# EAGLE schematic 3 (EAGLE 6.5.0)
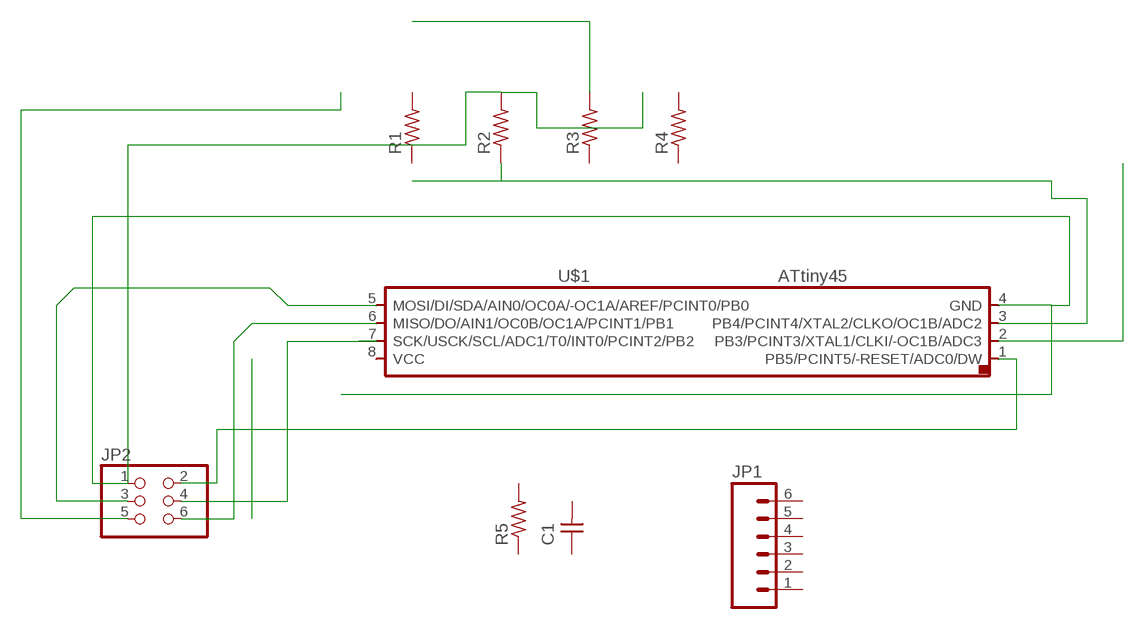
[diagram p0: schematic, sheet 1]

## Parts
C1  UNPOLARIZED_CAPACITOR1206  [1206]
JP1  M06SMD  [1X06-SMD]
JP2  PINHD-2X3-SMD  [2X03SMD]
R1  RESISTOR1206  [1206]
R2  RESISTOR1206  [1206]
R3  RESISTOR1206  [1206]
R4  RESISTOR1206  [1206]
R5  RESISTOR1206  [1206]
U$1  ATTINY45SI  [SOIC8]

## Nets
N$1: JP2.3 U$1.5(MOSI/DI/SDA/AIN0/OC0A/-OC1A/AREF/PCINT0/PB0)
N$2: JP2.5
N$3: JP2.2 U$1.1(PB5/PCINT5/-RESET/ADC0/DW)
N$5: JP2.4 U$1.7(SCK/USCK/SCL/ADC1/T0/INT0/PCINT2/PB2)
N$6: JP2.6 U$1.6(MISO/DO/AIN1/OC0B/OC1A/PCINT1/PB1)
N$8: R2.1 U$1.3(PB4/PCINT4/XTAL2/CLKO/OC1B/ADC2)
N$9: U$1.2(PB3/PCINT3/XTAL1/CLKI/-OC1B/ADC3)
N$10: JP2.1 R2.2 U$1.4(GND)
N$18: R3.2
Unconnected: C1.1 C1.2 JP1.1 JP1.2 JP1.3 JP1.4 JP1.5 JP1.6 R1.1 R1.2 R3.1 R4.1 R4.2 R5.1 R5.2 U$1.8(VCC)

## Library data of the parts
C1 = 01_FAB_Hello:UNPOLARIZED_CAPACITOR: unpolarized_capacitor
JP1 = 01_SparkFun:M06: Header 6 Standard 6-pin 0.1" header. Use with straight break away headers (SKU : PRT-00116), right angle break away headers (PRT-00553), swiss pins (PRT-00743), machine pins (PRT-00117), and female headers (PRT-00115). Molex polarized connector foot print use with SKU : PRT-08094 with associated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
JP2 = 01_FAB_Hello:PINHD-2X3-SMD: PIN HEADER
R1-R3 = ng:RESISTOR
R4 R5 = 01_ng:RESISTOR
U$1 = 01_fab:ATTINY45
